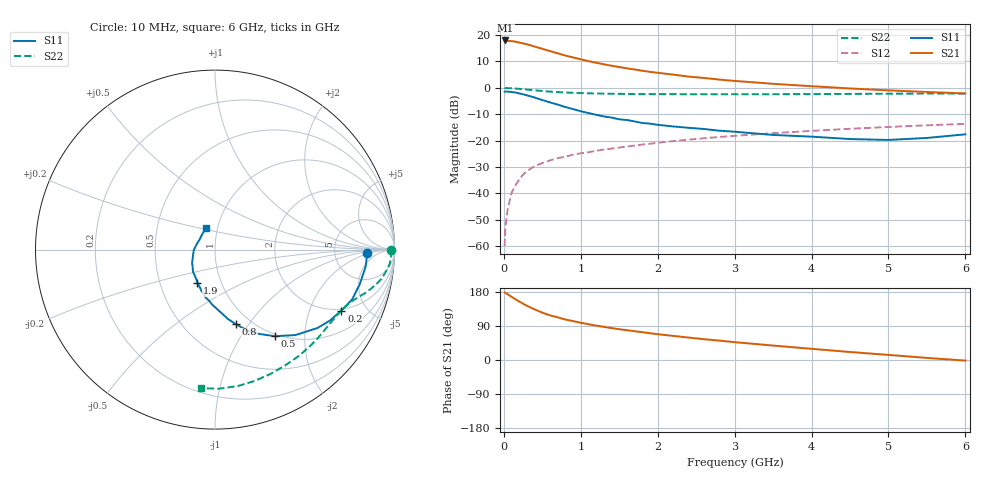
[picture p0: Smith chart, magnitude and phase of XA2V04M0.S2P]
! SIEMENS Discrete & RF Semiconductors
! BFY180
! Si NPN RF Bipolar Junction Transistor in MICRO-X
! VCE = 2 V  IC = 4 mA
! Common Emitter S-Parameters:  May  1997
# GHz  S  MA  R  50
!  f  S11  S21  S12  S22
! GHz  MAG  ANG  MAG  ANG  MAG  ANG  MAG  ANG
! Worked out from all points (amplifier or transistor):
!   36 points, 10 MHz to 6 GHz, reference 50 ohm
!   highest |S21| = 17.9 dB at 20 MHz (marker M1)
!   |S21| within 3 dB of that: start of sweep to 481.4 MHz
!   unconditionally stable (mu >= 1): 1.063 GHz to end of sweep
!   at 250 MHz: K = 0.33, MSG = 24.8 dB, |S12| = -32.9 dB
!   at 1.4 GHz: K = 1.13, MAG = 13.5 dB, |S12| = -23.0 dB
!   at 6 GHz: K = 1.19, MAG = 3.1 dB, |S12| = -13.7 dB
!   S11 on the Smith chart (normalised r, x): 10 MHz: 12, -2; 200 MHz: 1.91, -3.35; 500 MHz: 0.97, -1.42; 800 MHz: 0.85, -0.87; 1.9 GHz: 0.77, -0.30; 6 GHz: 0.88, +0.22
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0.01  0.8464 -1.4  7.745 178.5  0.001 87.3  0.9829 -0.2
0.02  0.8468 -2.9  7.862 177.1  0.0023 95.9  0.9834 -0.9
0.05  0.8445 -6.5  7.693 173.5  0.005 85.1  0.982 -2.2
0.1  0.8295 -13.4  7.647 166.9  0.0102 81.1  0.9772 -4.5
0.15  0.8133 -19.9  7.452 160.5  0.0141 78.4  0.9656 -6.6
0.2  0.7819 -25.8  7.19 154.4  0.0185 75.6  0.9522 -8.5
0.3  0.719 -37.4  6.652 143.0  0.0264 69.2  0.9226 -11.8
0.4  0.6535 -46.8  6.036 133.6  0.0327 65.4  0.8948 -14.2
0.5  0.5854 -55.5  5.464 125.1  0.0374 62.1  0.8674 -16.4
0.6  0.5279 -62.7  4.946 117.8  0.0422 59.8  0.8457 -18.0
0.8  0.4315 -74.3  4.065 106.9  0.0496 56.7  0.8128 -20.9
1  0.3591 -83.6  3.454 98.2  0.0574 55.2  0.7931 -23.6
1.1  0.3317 -88.0  3.189 94.4  0.0602 54.8  0.7844 -24.8
1.2  0.3077 -92.8  2.982 90.7  0.0639 53.9  0.7795 -26.2
1.5  0.2527 -104.2  2.468 81.2  0.0737 52.9  0.7662 -30.4
1.9  0.2092 -118.0  2 70.7  0.0869 50.9  0.7578 -36.1
2.2  0.1852 -126.8  1.774 63.7  0.0974 49.1  0.7559 -40.5
2.8  0.1538 -144.6  1.427 51.2  0.1168 45.8  0.7535 -49.0
3.5  0.1277 -163.8  1.188 38.1  0.138 40.9  0.7545 -58.9
4.5  0.1068 164.4  0.969 21.1  0.1671 33.4  0.7643 -73.2
5.5  0.1121 129.2  0.832 5.5  0.1944 25.5  0.7752 -88.1
6  0.1312 112.2  0.778 -1.6  0.207 21.3  0.7761 -95.6
